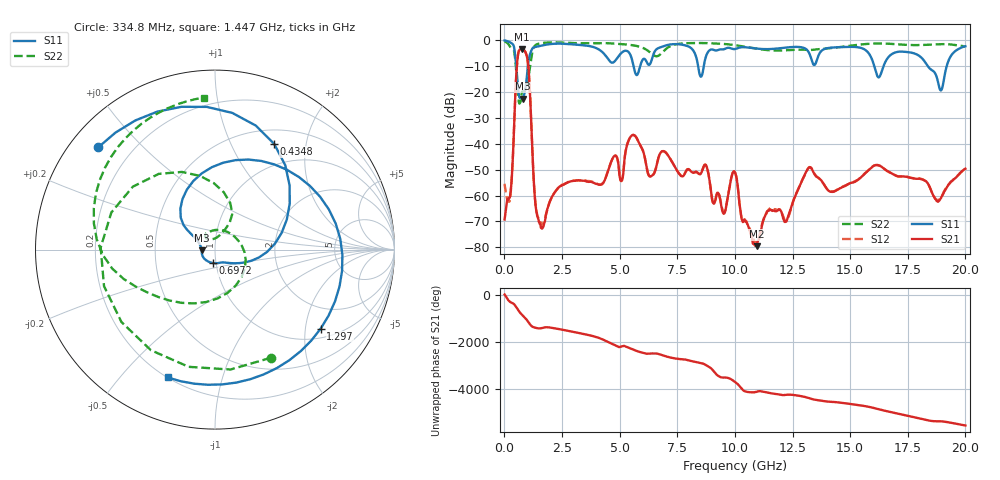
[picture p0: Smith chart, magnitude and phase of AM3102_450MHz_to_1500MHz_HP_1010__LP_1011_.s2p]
!Agilent Technologies,E8364B,MY43040894,A.07.50.67
!Agilent E8364B: A.07.50.67
!Date: Thursday, January 11, 2018 06:13:04
!Correction: S11(Full 2 Port(1,2))
!S21(Full 2 Port(1,2))
!S12(Full 2 Port(1,2))
!S22(Full 2 Port(1,2))
!S2P File: Measurements: S11, S21, S12, S22:
# Hz S  dB  R 50
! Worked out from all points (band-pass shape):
!   1601 points, 10 MHz to 20 GHz, reference 50 ohm
!   highest |S21| = -3.35 dB at 747.1 MHz (marker M1); lowest = -79.6 dB at 10.95 GHz (marker M2)
!   |S21| within 3 dB of the highest: 579.8 MHz to 978.7 MHz (398.9 MHz wide, 51.2 % of centre)
!   lowest |S11| = -22.6 dB at 797.1 MHz (marker M3), VSWR 1.16, Z = 43.1 - j0.255 ohm
!   |S11| at or under -10 dB: 514.9 MHz to 1.016 GHz (500.9 MHz wide, 65.4 % of centre); 16.05 GHz to 16.45 GHz (401.1 MHz wide, 2.47 % of centre); 18.37 GHz to 19.19 GHz (818 MHz wide, 4.36 % of centre)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
!   |S22| runs from -24.4 to -0.5 dB; largest |S21 - S12| = 0.0014
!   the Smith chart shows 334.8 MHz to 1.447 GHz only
!   S11 on the Smith chart (normalised r, x): 334.8 MHz: 0.08, +0.37; 434.8 MHz: 0.69, +1.48; 697.2 MHz: 0.97, -0.15; 1.297 GHz: 1.27, -2.43; 1.447 GHz: 0.20, -0.68
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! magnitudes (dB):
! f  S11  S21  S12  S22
! 10 MHz  -0.1  -69.3  -55.5  -0.5
! 334.8 MHz  -1.3  -51.1  -51.0  -3.4
! 434.8 MHz  -3.4  -29.8  -29.6  -4.8
! 697.2 MHz  -22.4  -3.4  -3.4  -23.8
! 747.1 MHz  -22.1  -3.3  -3.3  -20.8
! 797.1 MHz  -22.6  -3.4  -3.4  -19.8
! 1.034 GHz  -8.7  -9.9  -9.9  -14.9
! 1.297 GHz  -2.7  -57.6  -57.5  -2.3
! 1.447 GHz  -2.4  -68.4  -68.2  -1.4
! 3.346 GHz  -1.9  -54.3  -54.2  -1.1
! 5.082 GHz  -4.8  -54.4  -54.3  -1.5
! 5.57 GHz  -8.6  -36.6  -36.6  -1.9
! 6.307 GHz  -9.3  -52.7  -52.6  -4.6
! 6.682 GHz  -3.0  -45.5  -45.5  -6.0
! 8.731 GHz  -6.6  -48.1  -48.1  -1.1
! 9.518 GHz  -3.5  -67.1  -66.3  -1.4
! 10.01 GHz  -3.4  -51.0  -51.0  -1.9
! 10.95 GHz  -3.2  -79.6  -78.0  -3.3
! 13.34 GHz  -8.0  -49.8  -49.7  -3.7
! 16.68 GHz  -6.3  -50.8  -50.9  -1.3
! 18.94 GHz  -19.4  -61.0  -60.7  -1.5
! 20 GHz  -2.3  -49.6  -49.4  -2.4
